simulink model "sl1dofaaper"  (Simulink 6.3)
settings: Solver=ode3  SolverMode=SingleTasking  StartTime=0.0  StopTime=aat1  RelTol=1e-2  AbsTol=1e-3
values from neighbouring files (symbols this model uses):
  aadst1 = aadst1tmp    (= 0)    [aadata.m]    (also in runme.m = 100)
  aadsv1 = aadsv1tmp    (= 0)    [aadata.m]    (also in runme.m = 0.2)
  aarst1 = aarst1tmp    (= 0)    [aadata.m]    (also in runme.m = 1)
  aarsv1 = aarsv1tmp    (= 0)    [aadata.m]    (also in runme.m = 1)
  aat1 = aat1tmp    (= 0)    [aadata.m]    (also in runme.m = 200)
  m0 = 1    [runme.m]    (also in aaccpe.m = 0)
  m1 = 0    [runme.m]    (also in aaccpe.m)
  m2 = 0    [runme.m]    (also in aaccpe.m)
  m3 = 0    [runme.m]    (also in aaccpe.m)
  pStore = [1 1]    [runme.m]    (also in get_kp_td.m = p)
  qStore = [1 1]    [runme.m]    (also in get_kp_td.m = q)
  r0 = 1    [runme.m]    (also in aaccpe.m = 0)
  r1 = 0    [runme.m]    (also in aaccpe.m)
  r2 = 0    [runme.m]    (also in aaccpe.m)
  r3 = 0    [runme.m]    (also in aaccpe.m)
  Td = Tdtmp    (= 0)    [gsdata.m]    (also in runme.m = 4)

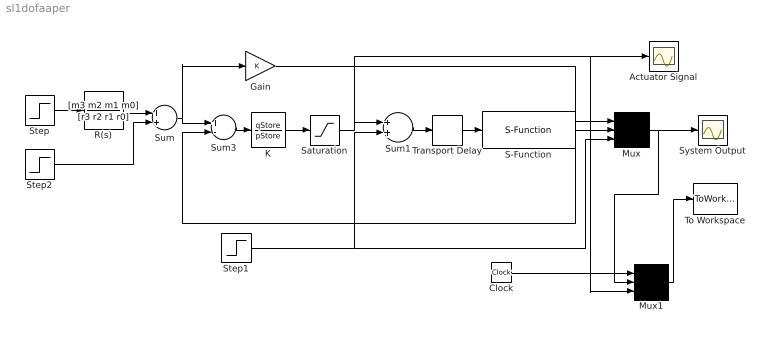
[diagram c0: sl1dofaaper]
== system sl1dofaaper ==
  Actuator Signal : Scope
  Clock : Clock
  Gain : Gain
  K : TransferFcn  Numerator=qStore  Denominator=pStore
  Mux : Mux  Inputs=3
  Mux1 : Mux  Inputs=3
  R(s) : TransferFcn  Numerator=[m3 m2 m1 m0]  Denominator=[r3 r2 r1 r0]
  S-Function : S-Function  FunctionName=sfperiodic
  Saturation : Saturate  UpperLimit=10  LowerLimit=-10
  Step : Step  Time=aarst1  After=aarsv1  SampleTime=0
  Step1 : Step  Time=400  After=0  SampleTime=0
  Step2 : Step  Time=aadst1  After=aadsv1  SampleTime=0
  Sum : Sum
  Sum1 : Sum
  Sum3 : Sum  Inputs=+-
  System Output : Scope
  To Workspace : ToWorkspace  VariableName=o7  SampleTime=aat1/10000  SaveFormat=Array
  Transport Delay : TransportDelay  DelayTime=Td  BufferSize=5000
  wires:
  Gain/1 -> Mux/1
  Sum1/1 -> Transport Delay/1
  Step1/1 -> Sum1/2, Mux/3
  Mux/1 -> System Output/1, Mux1/2
  Mux1/1 -> To Workspace/1
  Clock/1 -> Mux1/1
  Saturation/1 -> Sum1/1, Actuator Signal/1, Mux1/3
  S-Function/1 -> Mux/2, Sum3/2
  K/1 -> Saturation/1
  Step2/1 -> Sum/2
  Sum/1 -> Gain/1, Sum3/1
  Sum3/1 -> K/1
  Transport Delay/1 -> S-Function/1
  Step/1 -> R(s)/1
  R(s)/1 -> Sum/1
